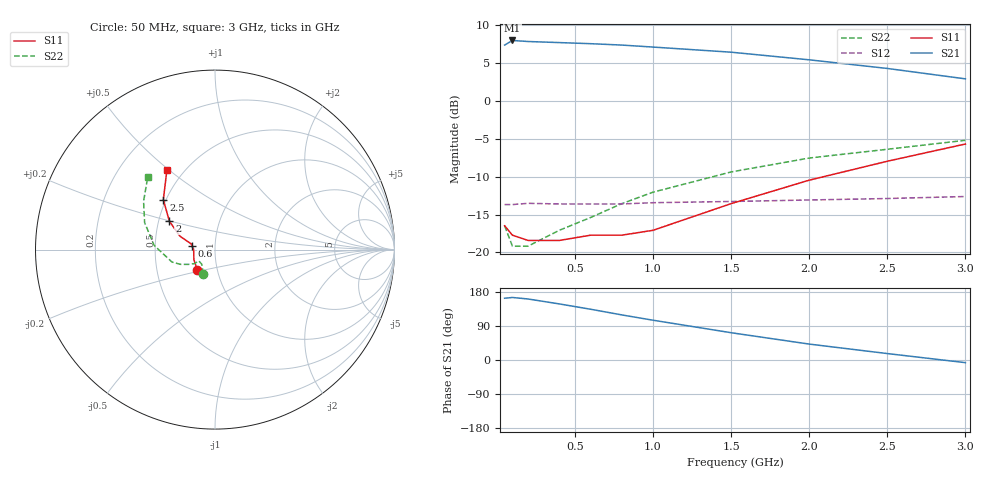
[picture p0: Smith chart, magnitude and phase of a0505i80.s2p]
!  MSA-0505 S PARAMETERS
!  Id=80 mA  LAST UPDATED 07-22-92
# ghz s ma r 50
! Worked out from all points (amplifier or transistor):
!   11 points, 50 MHz to 3 GHz, reference 50 ohm
!   highest |S21| = 8.0 dB at 100 MHz (marker M1)
!   |S21| within 3 dB of that: start of sweep to 2.194 GHz
!   unconditionally stable (mu >= 1): start of sweep to 2.65 GHz
!   at 100 MHz: K = 1.20, MAG = 8.2 dB, |S12| = -13.7 dB
!   at 800 MHz: K = 1.21, MAG = 7.7 dB, |S12| = -13.6 dB
!   at 3 GHz: K = 0.91, MSG = 7.8 dB, |S12| = -12.6 dB
!   S11 on the Smith chart (normalised r, x): 50 MHz: 0.80, -0.19; 600 MHz: 0.77, +0.03; 2 GHz: 0.57, +0.20; 2.5 GHz: 0.48, +0.32; 3 GHz: 0.40, +0.49
0.05  0.15 -131.0  2.34 163.0  0.207 7.0  0.15 -116.0
0.1  0.13 -155.0  2.51 165.0  0.207 3.0  0.11 -132.0
0.2  0.12 -170.0  2.47 161.0  0.211 1.0  0.11 -145.0
0.4  0.12 178.0  2.43 148.0  0.209 -1.0  0.14 -146.0
0.6  0.13 172.0  2.39 134.0  0.209 -2.0  0.17 -151.0
0.8  0.13 168.0  2.34 119.0  0.209 -3.0  0.21 -157.0
1  0.14 166.0  2.27 105.0  0.213 -4.0  0.25 -164.0
1.5  0.21 159.0  2.1 72.0  0.217 -6.0  0.34 176.0
2  0.3 148.0  1.87 42.0  0.222 -9.0  0.42 159.0
2.5  0.4 136.0  1.64 17.0  0.227 -11.0  0.48 146.0
3  0.52 121.0  1.4 -7.0  0.234 -16.0  0.55 133.0
